PROGRAM PRG_Recipe_TcPlcHMI	(*Twincat PLC HMI, 参数保存, 配方功能*)
VAR
	fbRecipeTcPlcHMI	: FB_Recipe_TcPlcHMI;
	eFileType			: E_FileType :=eFileType_BIN;
END_VAR


(*测试*)
VAR
	nErrorCounter			: INT;
	nDoneCounter			: INT;
END_VAR

;
fbRecipeTcPlcHMI(
	bRunOnCeDevice		:= FALSE,					(* TRUE--CE系统, FALSE--非CE系统*)
	sgFilePath			:= '\Data\Recipe\',			(* 文件路径, 默认是 \Data\Recipe\' *)
	eFileType			:= eFileType ,				(* 文件类型, 默认是XML, 只支持 eFileType_XML 和 eFileType_BIN 两种类型 *)
	pRecData			:= ADR(sRecData),			(* 配方参数首地址 *)
	pBakData			:= ADR(_sRecData),			(* 配方备份的首地址, 保存上一次的参数值, 用来比较参数是否有变化 *)
	nRecSize			:= SIZEOF(sRecData),		(* 配方总字节数 *)
	tAutoSaveRec		:= T#3S,					(* 参数变化后, 延时保存(写文件) *)
	sRecipeCtrl			:= g_sRecipeCtrl,			(* 触摸屏按钮, 配方名, 状态等等 *)
	bInitialDone		=> ,						(* 初始化完成 *)
	bDone				=> ,						(* 读写完成 *)
	bBusy				=> ,						(* 读写中 *)
	bError				=> ,						(* 读写失败 *)
	nErrorId			=> );						(* 错误代码 *)


(*测试*)
IF fbRecipeTcPlcHMI.bError THEN		(*没有作用, 要读取 LastResult.Error*)
	nErrorCounter := nErrorCounter + 1;
END_IF
IF fbRecipeTcPlcHMI.bDone THEN
	nDoneCounter := nDoneCounter + 1;
END_IF

END_PROGRAM
